

FUNCTION FC 2 : VOID
TITLE =Set transmission data for one specific SendDB


//Inputs are:
//OutputAddr    -> output bytes address range start
//InputAddr     -> input bytes address range start
//SrcDb         -> number of DB containing user data
//SendDb        -> number of SendDB assigned to display
//LenConsData   -> length of consistent data i.e. max length for one data segment
//
//Outputs:
//RETVAL:       -> = 0x0000 signals no error
VERSION : 0.1


VAR_INPUT
  OutputAddr : WORD ;	//first address of display outputs
  InputAddr : WORD ;	//address of display input
  SrcDb : WORD ;	//number of source DB (contains data to be sent)
  SendDb : WORD ;	//number of destination DB to be transmitted (also storage for TxHsByte)
  LenConsData : WORD ;	//number of consistent data bytes, MUST EQUAL LENGTH FOR CONFIGURED MODULE
END_VAR
VAR_OUTPUT
  RETVAL : INT ;	//0 if ok, error else (see description below)
END_VAR
VAR_TEMP
  T_DataLen : WORD ;	//number of bytes to be sent
  T_SEND : WORD ;	//temp storage for number of TxDB
  T_SRC : WORD ;	//temp storage for number of SrcDB
END_VAR
BEGIN
NETWORK
TITLE =
//open source DB and store transmission key data in SendDB

      L     W#16#0; // 0x0000 signals no error
      T     #RETVAL; // preset it here

      L     #SrcDb; // get number of source data block
      T     #T_SRC; // store locally
      AUF   DB [#T_SRC]; // open the SourceDB; must contain data string beginning in byte 0 of DB
      L     DBB    1; // string length saved in 2nd byte of string i.e byte 1 of source DB
      T     #T_DataLen; // store data length locally
      L     W#16#0; // load compare value
      ==I   ; // data length equals 0 ?
      SPB   ERR; // nothing to send; signal error and quit

      L     #LenConsData; // get number of specified output bytes
      L     W#16#0; // load compare value
      ==I   ; // length of output bytes specified with 0 ?
      SPB   ERR; // wrong input to function; signal error and quit

      L     #SendDb; // get number of SendDb
      T     #T_SEND; // store locally
      AUF   DB [#T_SEND]; // open the SendDb

      L     #T_DataLen; // get length of data to be sent
      L     #LenConsData; // get length of consistent data
      +     L#-1; // dec consistent data length by 1 (HsByte) to get max length for raw data
      /I    ; // div total data len by max len for raw data in one segment to get num of full segments
      T     DBW   64; // store in SendDb (SendDb.NumOfSegments)

      L     #T_DataLen; // get length of data to be sent
      L     #LenConsData; // get length of consistent data
      +     L#-1; // dec consistent data length by 1 (HsByte) to get max length for raw data
      MOD   ; // get remainder to find out if another segment must be sent
      L     W#16#0; // load 0
      ==I   ; // no remainder ?
      SPB   L110; // jump if true

      L     DBW   64; // get number of full segments (SendDb.NumOfSegments)
      +     1; // add 1 to send one more segment
      T     DBW   64; // store in SendDb (SendDb.NumOfSegments)

L110: NOP   0;
      L     W#16#0; // load value 0 (no segment sent)
      T     DBW   66; // store in SendDb (SendDb.SegmentCounter)

      L     #T_SRC; // load number of SourceDB (input to function)
      T     DBW   68; // store in SendDb (SendDb.SourceDB)

      L     #OutputAddr; // load address of display outputs (input to function)
      T     DBW   70; // store in SendDb (SendDb.OutputAddr)

      L     #InputAddr; // load address of display inputs (input to function)
      T     DBW   72; // store in SendDb (SendDb.InputAddr)

      L     #LenConsData; // load number of consistent data (input to function)
      T     DBW   74; // store in SendDb (SendDb.OutputLen)

      SPA   EXIT; // done, quit

NETWORK
TITLE =
//Leave with or without error

ERR:  NOP   0; // set error 0x0001 (error in data length)
      L     W#16#1;
      T     #RETVAL;
      SPA   EXIT; // leave with result = 0x0001

EXIT: NOP   0; // common exit point
      BE    ;


END_FUNCTION

